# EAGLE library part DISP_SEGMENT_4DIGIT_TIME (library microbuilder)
4-Digit 7-Segment Display with colon and AM/PM dots - Common Cathode
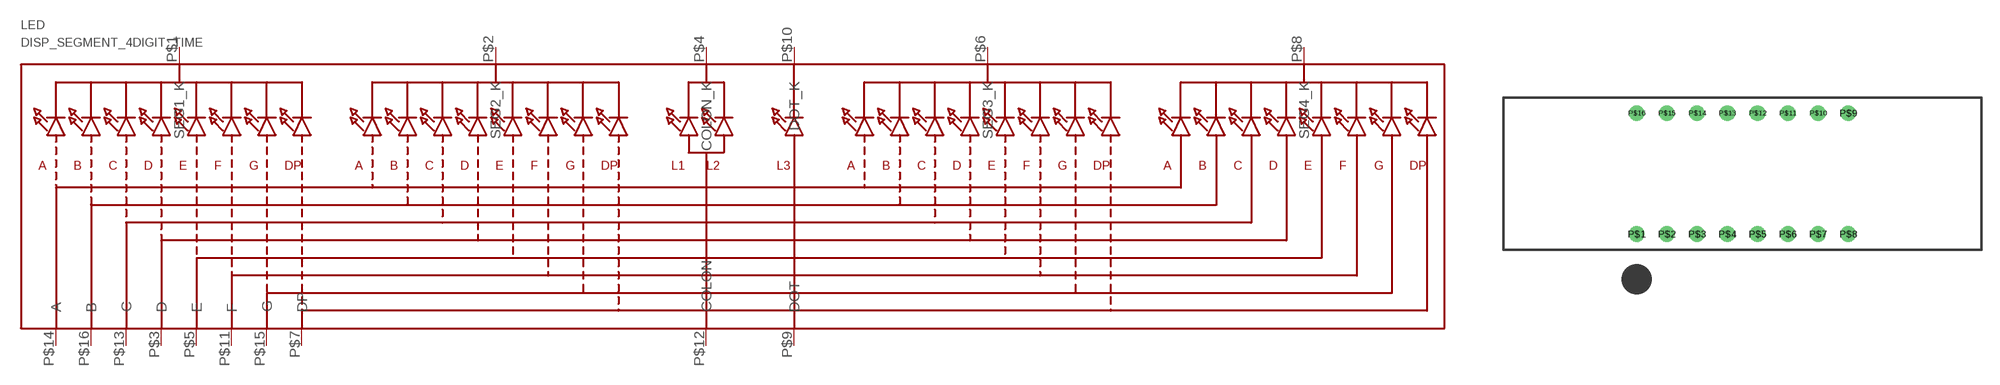
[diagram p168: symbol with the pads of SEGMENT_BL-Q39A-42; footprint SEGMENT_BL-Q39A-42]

Designator prefix LED

## DISP_SEGMENT_4DIGIT_TIME  [SEGMENT_BL-Q39A-42]
P$1  SEG1_K
P$2  SEG2_K
P$3  D
P$4  COLON_K
P$5  E
P$6  SEG3_K
P$7  DP
P$8  SEG4_K
P$9  DOT
P$10  DOT_K
P$11  F
P$12  COLON
P$13  C
P$14  A
P$15  G
P$16  B

## Footprint SEGMENT_BL-Q39A-42 (pad centres in mm)
drill 0.8: P$1 -8.89,-5.08; P$2 -6.35,-5.08; P$3 -3.81,-5.08; P$4 -1.27,-5.08; P$5 1.27,-5.08; P$6 3.81,-5.08; P$7 6.35,-5.08; P$8 8.89,-5.08; P$9 8.89,5.08; P$10 6.35,5.08; P$11 3.81,5.08; P$12 1.27,5.08; P$13 -1.27,5.08; P$14 -3.81,5.08; P$15 -6.35,5.08; P$16 -8.89,5.08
